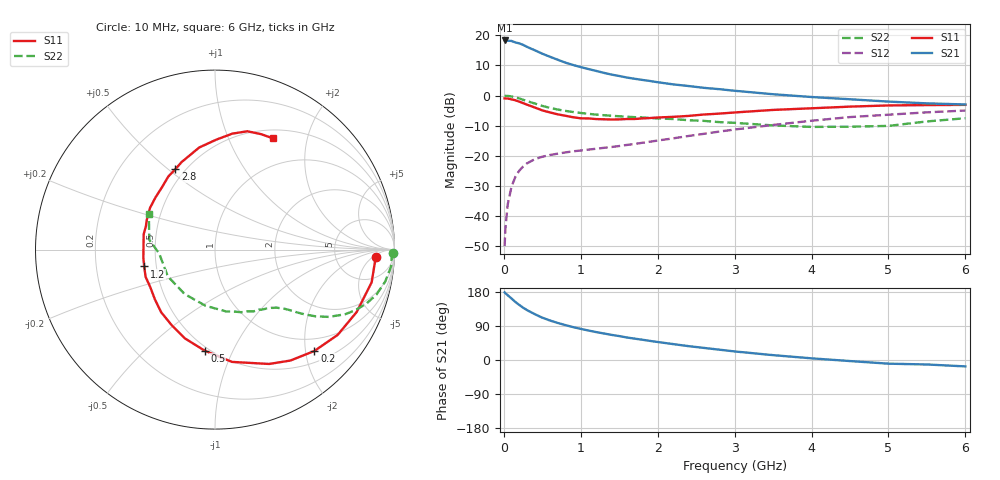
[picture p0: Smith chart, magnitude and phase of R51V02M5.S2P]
! SIEMENS Small Signal Semiconductors
! BFR183
! Si NPN RF Bipolar Junction Transistor in SOT23
! VCE = 1 V  IC = 2.5 mA
! Common Emitter S-Parameters:  May  1996
# GHz  S  MA  R  50
!  f  S11  S21  S12  S22
! GHz  MAG  ANG  MAG  ANG  MAG  ANG  MAG  ANG
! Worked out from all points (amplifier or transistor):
!   36 points, 10 MHz to 6 GHz, reference 50 ohm
!   highest |S21| = 18.3 dB at 10 MHz (marker M1)
!   |S21| within 3 dB of that: start of sweep to 378.4 MHz
!   unconditionally stable (mu >= 1): 1.27 GHz to 2.984 GHz
!   at 250 MHz: K = 0.27, MSG = 20.3 dB, |S12| = -23.7 dB
!   at 1.4 GHz: K = 1.06, MAG = 10.6 dB, |S12| = -17.1 dB
!   at 6 GHz: K = 0.94, MSG = 1.0 dB, |S12| = -5.0 dB
!   S11 on the Smith chart (normalised r, x): 10 MHz: 16, -6; 200 MHz: 0.72, -2.18; 500 MHz: 0.47, -0.78; 1.2 GHz: 0.43, -0.10; 2.8 GHz: 0.44, +0.53; 6 GHz: 0.61, +1.47
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0.01  0.8957 -2.5  8.255 178.5  0.0031 87.2  0.9939 -1.0
0.02  0.8932 -4.9  8.148 176.3  0.006 85.6  0.9853 -2.1
0.05  0.8917 -11.8  8.179 171.0  0.0153 82.2  0.9856 -5.5
0.1  0.8625 -23.8  8.094 162.3  0.0305 76.9  0.9647 -10.7
0.15  0.8325 -34.8  7.647 153.1  0.0442 70.8  0.9335 -15.6
0.2  0.7909 -45.6  7.384 145.4  0.0559 66.0  0.8952 -19.7
0.25  0.7474 -55.8  6.975 138.0  0.0656 61.0  0.8498 -23.5
0.3  0.7048 -64.7  6.464 131.8  0.074 57.6  0.8098 -26.4
0.4  0.6328 -81.4  5.684 121.2  0.0869 51.4  0.7367 -30.6
0.5  0.5658 -95.9  4.969 111.7  0.0956 47.5  0.6715 -33.6
0.6  0.5223 -108.7  4.417 104.3  0.1023 45.0  0.6221 -35.6
0.7  0.486 -119.6  3.941 97.8  0.1075 43.7  0.5843 -37.1
0.8  0.4601 -130.7  3.532 92.1  0.1128 42.5  0.5548 -38.2
1.1  0.4153 -158.6  2.758 77.8  0.1257 42.8  0.4952 -41.4
1.2  0.4055 -166.6  2.566 73.7  0.1299 43.3  0.4813 -42.5
1.6  0.4065 167.7  1.992 59.4  0.1503 46.1  0.4434 -47.4
2.2  0.4412 138.6  1.533 42.0  0.1933 49.0  0.406 -57.9
2.8  0.4995 116.2  1.276 27.3  0.2509 47.9  0.3607 -73.1
3.5  0.5755 98.8  1.05 12.8  0.3234 42.2  0.3177 -99.3
4.5  0.6532 81.5  0.866 -2.8  0.4374 29.8  0.3023 -150.4
5.5  0.6927 68.1  0.74 -11.8  0.5247 16.5  0.37 171.6
6  0.6986 62.6  0.709 -16.9  0.562 7.8  0.4187 151.7
